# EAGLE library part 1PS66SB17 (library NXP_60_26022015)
4 V, 30 mA low Cd Schottky barrier diode Planar low capacitance Schottky barrier diode encapsulated in a very small SMD plastic package. AAL Eindhoven MK
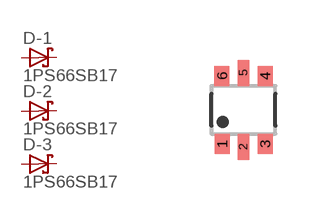
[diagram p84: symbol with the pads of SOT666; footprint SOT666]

Designator prefix D; gates -1=DIODE_SCHOTTKY -2=DIODE_SCHOTTKY -3=DIODE_SCHOTTKY

## 1PS66SB17  [SOT666]
1  -1:A  pas
2  -2:A  pas
3  -3:A  pas
4  -3:K  pas
5  -2:K  pas
6  -1:K  pas

## Footprint SOT666 (pad centres in mm)
SOT 666 Reflow soldering foorprint Source: Philips - BAS70_1PS7XSB70_SER_8.pdf
smd 0.375 x 0.5: 1 -0.537,-0.85; 3 0.538,-0.85; 4 0.538,0.85; 6 -0.538,0.85
smd 0.3 x 0.65: 2 0,-0.925; 5 0,0.925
